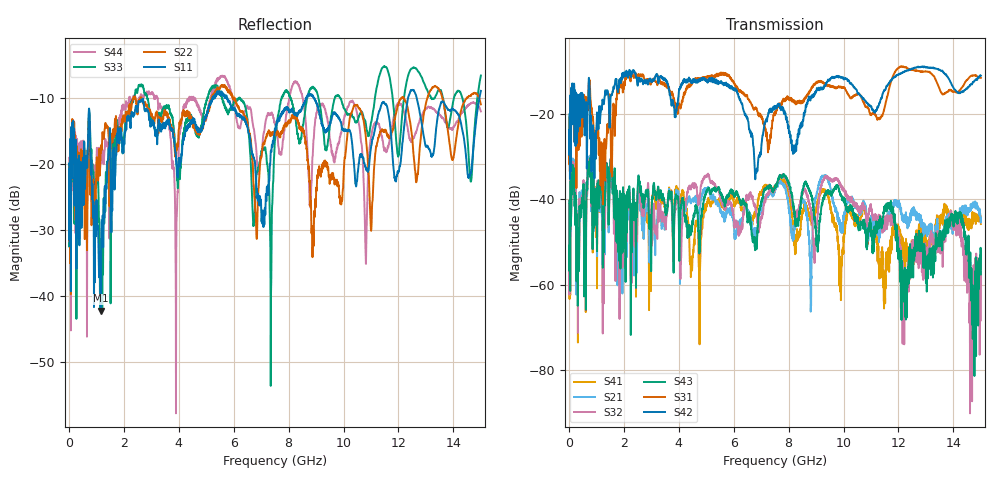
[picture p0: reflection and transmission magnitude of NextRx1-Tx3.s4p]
! FILE: N:\QM 2007\Prüfprotokolle\Highspeed\Konfektionierte Ltg\L45593-D106\D30\8216\0002\Next\NextRx1-Tx3.s4p
# MHz S DB R 50.00
! FREQ  S11  S12  S13  S14
!  S21  S22  S23  S24
!  S31  S32  S33  S34
!  S41  S42  S43  S44
!  DB  ANG  DB  ANG  DB  ANG  DB  ANG
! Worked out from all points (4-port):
!   2999 points, 10 MHz to 15 GHz, reference 50 ohm
!   strongest paths, dB at 10 MHz, 3.755 GHz, 7.505 GHz, 11.26 GHz, 15 GHz:
!     S42: -23.9, -17.0, -18.6, -18.5, -11.0
!     S31: -23.9, -14.8, -20.2, -21.0, -11.5
!     S43: -53.6, -40.6, -36.9, -46.7, -57.6
!     S32: -45.5, -41.6, -37.0, -45.0, -68.3
!     S21: -56.5, -43.4, -38.0, -47.5, -44.5
!     S41: -54.7, -42.3, -37.0, -50.5, -45.8
!   lowest |S11| = -42.2 dB at 1.16 GHz (marker M1), VSWR 1.02, Z = 49.3 + j0.321 ohm
!   |S11| at or under -10 dB: start of sweep to 5.225 GHz; 5.748 GHz to 8.654 GHz (2.907 GHz wide, 40.4 % of centre); 8.921 GHz to 12.35 GHz (3.428 GHz wide, 32.2 % of centre)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
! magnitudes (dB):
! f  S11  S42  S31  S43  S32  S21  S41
! 10 MHz  -19.9  -23.9  -23.9  -53.6  -45.5  -56.5  -54.7
! 1.16 GHz  -42.2  -19.7  -36.0  -37.6  -38.6  -41.4  -39.8
! 2.595 GHz  -10.6  -12.5  -11.1  -38.1  -40.3  -42.7  -40.3
! 7.355 GHz  -18.0  -19.5  -25.6  -36.9  -37.7  -38.6  -37.0
! 7.88 GHz  -11.8  -19.8  -16.4  -34.4  -34.5  -37.2  -36.0
! 11.5 GHz  -10.9  -14.5  -18.5  -42.7  -47.2  -46.5  -60.4
! 15 GHz  -9.0  -11.0  -11.5  -57.6  -68.3  -44.5  -45.8
